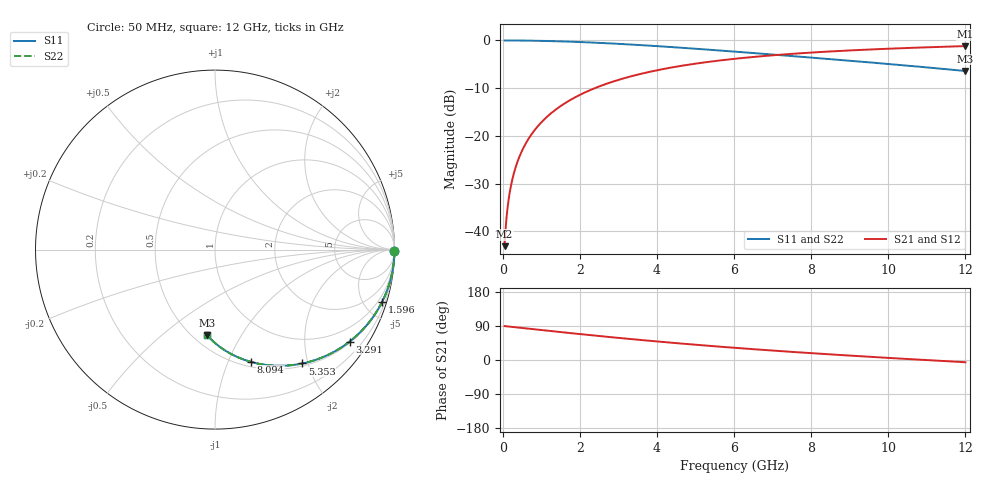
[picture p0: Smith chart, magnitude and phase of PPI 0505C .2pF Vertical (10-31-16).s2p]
# GHz S MA R 50
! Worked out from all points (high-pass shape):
!   1601 points, 50 MHz to 12 GHz, reference 50 ohm
!   highest |S21| = -1.18 dB at 12 GHz (marker M1); lowest = -43.1 dB at 50 MHz (marker M2)
!   |S21| within 3 dB of the highest: 5.641 GHz to end of sweep
!   lowest |S11| = -6.4 dB at 12 GHz (marker M3), VSWR 2.83, Z = 29.3 - j36.2 ohm
!   |S11| at or under -10 dB: nowhere
!   |S22| runs from -6.4 to 0.0 dB; largest |S21 - S12| = 0
!   S11 on the Smith chart (normalised r, x): 50 MHz: open; 1.596 GHz: 0.54, -6.53; 3.291 GHz: 0.54, -3.15; 5.353 GHz: 0.54, -1.91; 8.094 GHz: 0.55, -1.21; 12 GHz: 0.59, -0.72
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0.05  1 -0.5  0.006982 89.5  0.006982 89.5  1 -0.5
0.079875  0.9999 -0.9  0.01115 89.1  0.01115 89.1  0.9999 -0.9
0.1470937  0.9998 -1.6  0.02053 88.4  0.02053 88.4  0.9998 -1.6
0.1844375  0.9997 -2.0  0.02574 88.0  0.02574 88.0  0.9997 -2.0
0.2217813  0.9995 -2.4  0.03095 87.6  0.03095 87.6  0.9995 -2.4
0.2740625  0.9992 -3.0  0.03824 87.0  0.03824 87.0  0.9992 -3.0
0.3338125  0.9989 -3.7  0.04656 86.3  0.04656 86.3  0.9989 -3.7
0.4831875  0.9977 -5.3  0.06731 84.7  0.06731 84.7  0.9977 -5.3
0.6848437  0.9954 -7.5  0.09518 82.5  0.09518 82.5  0.9954 -7.5
0.9313125  0.9916 -10.2  0.1289 79.8  0.1289 79.8  0.9916 -10.2
1.237531  0.9853 -13.5  0.1702 76.5  0.1702 76.5  0.9853 -13.5
1.596031  0.9759 -17.3  0.2174 72.7  0.2174 72.7  0.9759 -17.3
2.044156  0.9613 -22.0  0.2742 68.0  0.2742 68.0  0.9613 -22.0
2.61925  0.9388 -27.8  0.3431 62.1  0.3431 62.1  0.9388 -27.8
3.291437  0.9082 -34.4  0.4169 55.5  0.4169 55.5  0.9082 -34.4
4.038312  0.8705 -41.3  0.4902 48.6  0.4902 48.6  0.8705 -41.3
5.352812  0.7999 -52.5  0.5976 37.4  0.5976 37.4  0.7999 -52.5
6.025  0.7635 -57.7  0.6429 32.1  0.6429 32.1  0.7635 -57.7
8.019156  0.6604 -71.8  0.7472 17.9  0.7472 17.9  0.6604 -71.8
8.093844  0.6567 -72.3  0.7504 17.4  0.7504 17.4  0.6567 -72.3
10.01331  0.5661 -84.1  0.8196 5.5  0.8196 5.5  0.5661 -84.1
12  0.4782 -95.3  0.8725 -5.9  0.8725 -5.9  0.4782 -95.3
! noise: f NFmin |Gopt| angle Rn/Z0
0.05  0.004112  0.993  0.5428  0.1356
1.372  0.006665  0.8437  10.03  0.008983
2.701  0.009295  0.7584  15.01  0.007657
4.031  0.01178  0.7068  18.88  0.007689
5.36  0.01417  0.6727  22.41  0.008031
6.682  0.01649  0.6489  25.78  0.008494
8.012  0.01883  0.6319  29.09  0.009034
9.341  0.02119  0.62  32.31  0.009639
10.67  0.02361  0.6122  35.47  0.01031
12  0.02613  0.6076  38.54  0.01106
